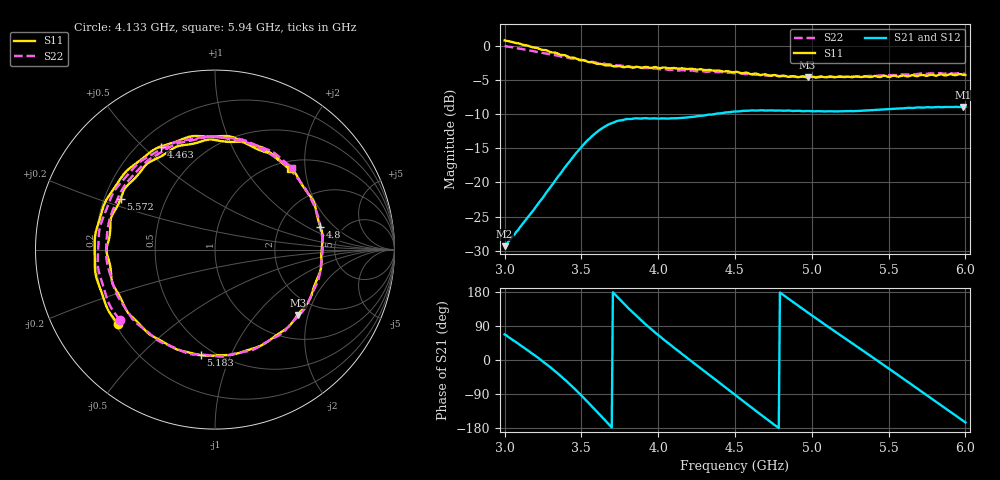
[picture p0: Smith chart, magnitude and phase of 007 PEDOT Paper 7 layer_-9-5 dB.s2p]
!  04/11/2025  19:38:23
! Ref Plane: 0.000 mm
# MHZ S MA R  50
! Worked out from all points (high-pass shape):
!   401 points, 3 GHz to 6 GHz, reference 50 ohm
!   highest |S21| = -8.93 dB at 5.985 GHz (marker M1); lowest = -29.3 dB at 3 GHz (marker M2)
!   |S21| within 3 dB of the highest: 3.646 GHz to end of sweep
!   lowest |S11| = -4.6 dB at 4.973 GHz (marker M3), VSWR 3.84, Z = 77.5 - j85.9 ohm
!   |S11| at or under -10 dB: nowhere
!   |S22| runs from -4.6 to 0.0 dB; largest |S21 - S12| = 0.0079
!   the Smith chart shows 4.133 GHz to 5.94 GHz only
!   S11 on the Smith chart (normalised r, x): 4.133 GHz: 0.21, -0.32; 4.463 GHz: 0.29, +0.57; 4.8 GHz: 3.44, +1.35; 5.183 GHz: 0.43, -0.78; 5.572 GHz: 0.27, +0.24; 5.94 GHz: 1.16, +1.66
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3000  1.095 -113.5  0.03418 67.7  0.03442 68.8  0.9981 -117.4
3270  0.9282 179.4  0.08389 -10.2  0.08396 -9.1  0.8797 175.6
3502.5  0.7881 100.8  0.1833 -94.7  0.1835 -94.2  0.7832 95.9
3607.5  0.7374 56.8  0.2374 -138.9  0.2378 -138.6  0.7468 52.6
3735  0.71 0.1  0.2821 165.9  0.2826 166.8  0.7189 -2.5
3862.5  0.7023 -52.2  0.2946 114.6  0.2962 115.7  0.6972 -53.8
4005  0.6872 -102.3  0.2935 64.4  0.2933 65.2  0.6752 -103.3
4132.5  0.6803 -142.8  0.296 23.4  0.2969 24.3  0.6597 -143.7
4290  0.6691 169.8  0.3078 -26.3  0.3082 -25.2  0.6525 167.6
4462.5  0.6489 117.7  0.3265 -80.0  0.3278 -79.0  0.6376 112.9
4500  0.6433 105.2  0.3308 -91.9  0.3326 -91.2  0.6293 100.9
4635  0.6272 63.5  0.3357 -133.9  0.3363 -133.3  0.614 57.4
4800  0.6008 12.1  0.3361 175.9  0.336 176.8  0.6017 5.9
4972.5  0.5868 -38.3  0.3335 125.6  0.3331 126.4  0.5922 -45.4
5002.5  0.5938 -46.8  0.3319 117.2  0.3314 117.9  0.596 -53.5
5182.5  0.5931 -97.6  0.3317 66.5  0.3314 67.1  0.5985 -103.9
5505  0.5921 171.2  0.3449 -23.5  0.3463 -22.5  0.61 167.2
5572.5  0.5972 151.6  0.3486 -42.7  0.3504 -41.6  0.6156 148.2
5767.5  0.6115 95.3  0.355 -98.5  0.3562 -97.5  0.6289 94.2
5940  0.6109 47.0  0.3573 -147.7  0.3587 -146.8  0.6273 46.7
5985  0.6136 35.4  0.3577 -160.1  0.3593 -159.4  0.6244 35.0
6000  0.6115 30.5  0.3573 -164.7  0.3583 -164.0  0.6239 30.3
